TYPE UDT 2

  STRUCT
   ChanA : ARRAY [1 .. 8] OF STRUCT 	//From Channel 1 to Channel 10
    FDD_5C00xx : ARRAY  [0 .. 15 ] OF //Feed disable A.no.51000-510015
    BOOL ;
    FDD_RID_5C01xx : ARRAY  [0 .. 31 ] OF //Feed and read-in disable A.no.510100-510131
    BOOL ;
    RID_5C02xx : ARRAY  [0 .. 31 ] OF //Read-in disable A.no.510200-510231
    BOOL ;
    NCSD_5C03xx : ARRAY  [0 .. 15 ] OF //NC start disable A.no.510300-510315
    BOOL ;
    FdStop_1_5C11xx : ARRAY  [0 .. 15 ] OF //Feed stop GEOaxis 1 A.no.511100-511115
    BOOL ;
    FdStop_2_5C12xx : ARRAY  [0 .. 15 ] OF //Feed stop GEOaxis 2 A.no.511200-511215
    BOOL ;
    FdStop_3_5C13xx : ARRAY  [0 .. 15 ] OF //Feed stop GEOaxis 3 A.no.511300-511315
    BOOL ;
   END_STRUCT ;
//Alarmno for Chan are 5Cxxxx; C is the ChannelNo, except Channel 10. Channel 10 has a value C = 0
    AxisA : ARRAY [1 .. 18] OF STRUCT  //From Axis 1 to Axis 31
    AAFdStop60AAxx : ARRAY  [0 .. 15 ] OF //Feed stop axis/spindle
    BOOL ;
   END_STRUCT ;
//Alarmno for Axis are 60AAxx; A is the Axisno.
   UserA : ARRAY [0 .. 63] OF STRUCT
   A70UUxx : ARRAY  [0 .. 63 ] OF //Alarm 700000-700063 (user area 0)
   BOOL ;
   END_STRUCT ;
//Alarmno for UserAlarms are 7yUUxx; U is the Userarea, y = Db1004.UserDek2No[U]
  END_STRUCT ;
END_TYPE

